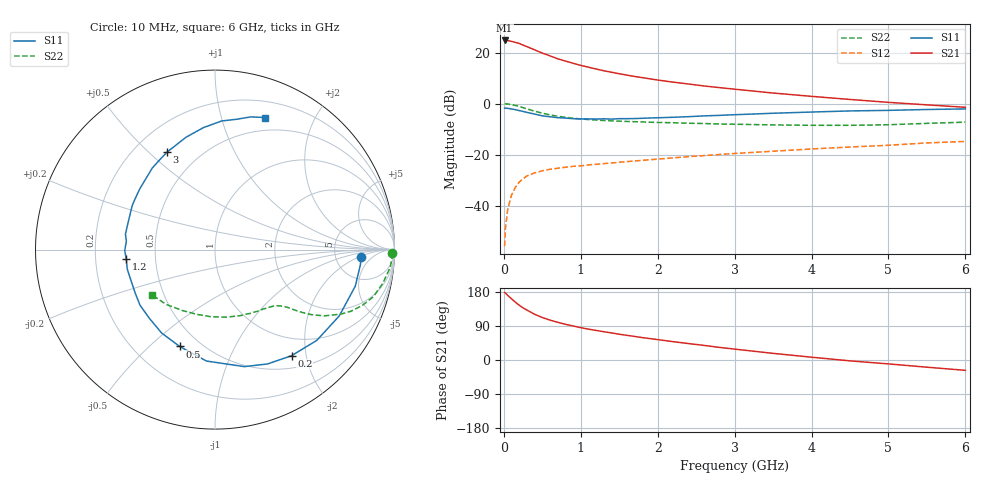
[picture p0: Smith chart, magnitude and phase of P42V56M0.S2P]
! SIEMENS Small Signal Semiconductors
! BFP182
! Si NPN RF Bipolar Junction Transistor in SOT143
! VCE = 2.5 V  IC = 6 mA
! Common Emitter S-Parameters:  March  1996
# GHz  S  MA  R  50
!  f  S11  S21  S12  S22
! GHz  MAG  ANG  MAG  ANG  MAG  ANG  MAG  ANG
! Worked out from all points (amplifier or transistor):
!   36 points, 10 MHz to 6 GHz, reference 50 ohm
!   highest |S21| = 24.8 dB at 10 MHz (marker M1)
!   |S21| within 3 dB of that: start of sweep to 345.7 MHz
!   unconditionally stable (mu >= 1): 1.453 GHz to 5.446 GHz
!   at 250 MHz: K = 0.24, MSG = 26.2 dB, |S12| = -29.5 dB
!   at 1.4 GHz: K = 0.99, MSG = 17.8 dB, |S12| = -23.3 dB
!   at 6 GHz: K = 0.93, MSG = 6.7 dB, |S12| = -14.8 dB
!   lowest NFmin = 1.25 dB at 450 MHz
!   S11 on the Smith chart (normalised r, x): 10 MHz: 9.19, -2.33; 200 MHz: 0.69, -1.74; 500 MHz: 0.39, -0.63; 1.2 GHz: 0.34, -0.05; 3 GHz: 0.33, +0.57; 6 GHz: 0.36, +1.38
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0.01  0.8145 -3.0  17.29 178.2  0.0016 91.2  0.9883 -1.2
0.02  0.8146 -5.9  17.24 176.6  0.0035 83.9  0.9886 -2.3
0.05  0.8077 -14.6  17.2 170.5  0.0084 83.9  0.9812 -5.8
0.1  0.7847 -28.1  16.6 161.4  0.0161 73.7  0.9533 -11.4
0.15  0.7601 -41.7  15.85 152.6  0.0228 68.1  0.9213 -16.5
0.2  0.7289 -54.2  15.11 144.5  0.0289 63.3  0.8784 -20.7
0.25  0.7012 -65.3  14.04 137.5  0.0335 59.0  0.8316 -24.4
0.3  0.6722 -75.9  13.08 131.8  0.0381 54.7  0.7872 -27.2
0.4  0.6227 -94.4  11.32 120.7  0.0438 48.8  0.7107 -31.3
0.5  0.5745 -110.0  9.786 112.1  0.0481 43.2  0.6482 -34.0
0.6  0.5517 -122.6  8.631 105.2  0.0515 41.2  0.6009 -35.7
0.7  0.5296 -133.5  7.562 99.5  0.0539 39.2  0.5653 -36.9
0.8  0.5201 -143.5  6.828 94.2  0.0564 38.0  0.5392 -37.8
1.1  0.5007 -167.6  5.171 81.4  0.0629 36.4  0.486 -40.3
1.2  0.4972 -173.9  4.758 78.0  0.0644 36.2  0.4756 -41.3
1.7  0.5089 160.2  3.401 62.2  0.0749 36.2  0.4409 -46.7
2.2  0.5389 141.0  2.634 48.4  0.0863 36.0  0.4214 -54.0
3  0.6053 116.2  1.917 28.7  0.1051 33.3  0.394 -69.1
3.5  0.6463 104.5  1.61 17.5  0.1164 30.8  0.3817 -80.2
4.5  0.7177 87.0  1.205 -2.3  0.1408 25.3  0.3747 -105.5
5.5  0.7659 74.9  0.944 -19.0  0.1693 19.3  0.4092 -131.7
6  0.7862 69.4  0.846 -27.3  0.1813 14.9  0.4323 -144.4
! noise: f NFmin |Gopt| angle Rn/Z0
0.45  1.25  0.25  39  0.3
0.9  1.4  0.25  78  0.23
1.8  1.95  0.21  151  0.2
